PROGRAM MAIN
VAR
	fbFileCopy : FB_FileCopy;
	fbFindFile : FB_EnumFindFileEntry; (* File search *)

	bCopy: BOOL;
END_VAR

fbFileCopy(
	bExecute := bCopy, 
	sSrcNetId:= '',
	sSrcPathName:= 'c:\temp\settings.txt',
	sDestNetId:= '',
	sDestPathName:= 'd:\temp\Newsettings001.txt', tTimeOut := T#5S);
	
PRG_FileFindEnumList();

END_PROGRAM
